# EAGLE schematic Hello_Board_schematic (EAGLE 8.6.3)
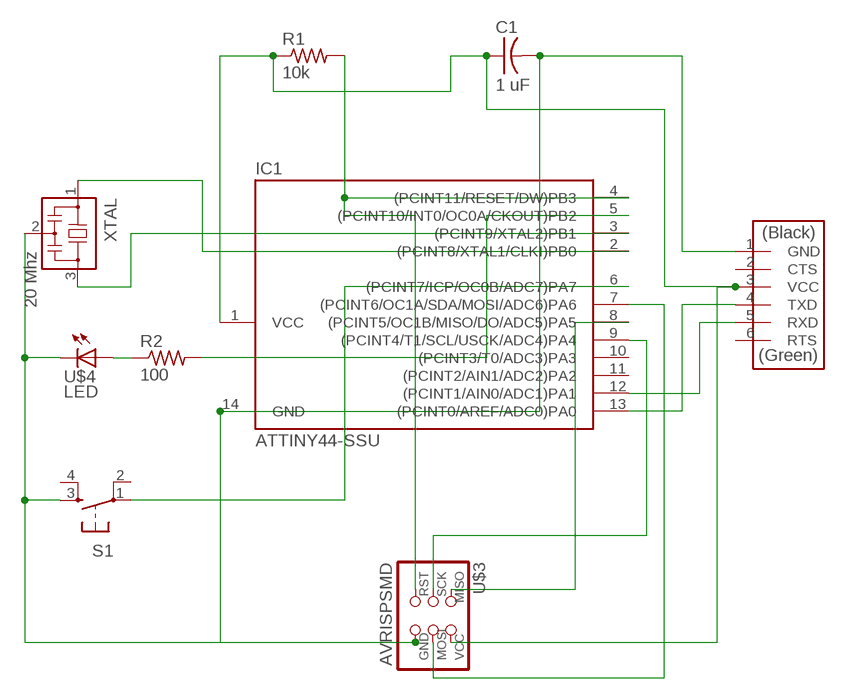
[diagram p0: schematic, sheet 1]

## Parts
C1  1 uF  CAP-US1206K  [C1206K]
IC1  ATTINY44-SSU  [SOIC14]
R1  10k  RES-US1206FAB  [R1206FAB]
R2  100  RES-US1206FAB  [R1206FAB]
S1  6MM_SWITCH6MM_SWITCH  [6MM_SWITCH]
U$2  FTDI-SMD-HEADER  [1X06SMD]
U$3  AVRISPSMD  [2X03SMD]
U$4  LED  [LED1206]
XTAL  20 Mhz  RESONATOR  [EFOBM]

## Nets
N$1: IC1.2((PCINT8/XTAL1/CLKI)PB0) XTAL.1
N$2: IC1.3((PCINT9/XTAL2)PB1) XTAL.3
N$3: C1.2 IC1.14(GND) S1.3(S) U$2.1(GND) U$3.6(GND) U$4.2(C) XTAL.2
N$4: IC1.4((PCINT11/RESET/DW)PB3) R1.2 U$3.5(RST)
N$5: IC1.5((PCINT10/INT0/OC0A/CKOUT)PB2) R2.2
N$6: C1.1 IC1.1(VCC) R1.1 U$2.3(VCC) U$3.2(VCC)
N$7: R2.1 U$4.1(A)
N$8: IC1.7((PCINT6/OC1A/SDA/MOSI/ADC6)PA6) U$3.4(MOSI)
N$9: IC1.9((PCINT4/T1/SCL/USCK/ADC4)PA4) U$3.3(SCK)
N$10: IC1.8((PCINT5/OC1B/MISO/DO/ADC5)PA5) U$3.1(MISO)
N$11: IC1.12((PCINT1/AIN0/ADC1)PA1) U$2.5(RXD)
N$12: IC1.13((PCINT0/AREF/ADC0)PA0) U$2.4(TXD)
N$13: IC1.6((PCINT7/ICP/OC0B/ADC7)PA7) S1.1(P)
Unconnected: IC1.10((PCINT3/T0/ADC3)PA3) IC1.11((PCINT2/AIN1/ADC2)PA2) S1.2(P1) S1.4(S1) U$2.2(CTS) U$2.6(RTS)

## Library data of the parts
C1 = fab:CAP-US
IC1 = fab:ATTINY44
R1 R2 = fab:RES-US: Resistor (US Symbol)
S1 = fab:6MM_SWITCH: OMRON SWITCH
U$2 = fab:FTDI-SMD-HEADER
U$3 = fab:AVRISP
U$4 = fab:LED: LED
XTAL = fab:RESONATOR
